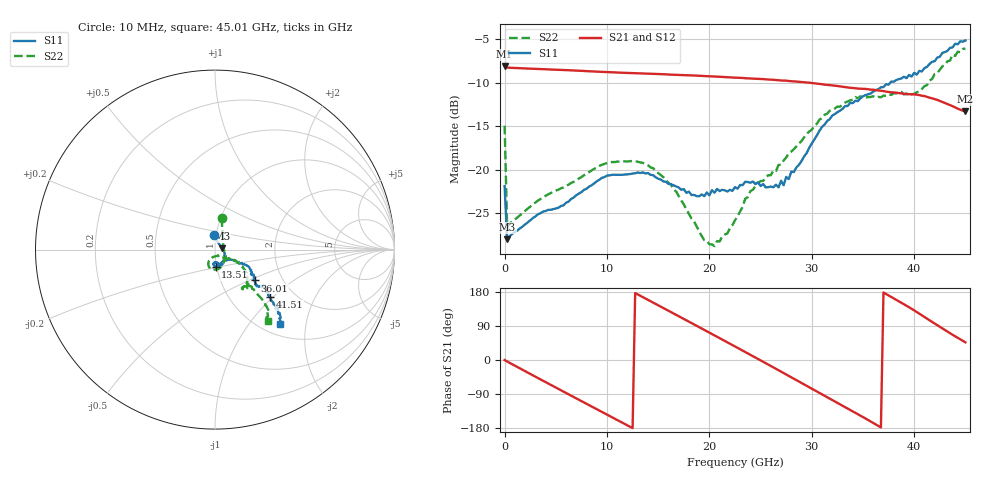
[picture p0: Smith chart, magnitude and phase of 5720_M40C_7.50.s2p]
! Device:  ADRF5720
! Description: 0.5dB LSB GaAs MMIC 6-bit Digital Attenuator
! Frequency:  0.000009 -  40 GHz
! Ports:
!	RF1	= Port 1
!	RF2	= Port 2
! Vdd:  3.3 Volt
! Vss:  -3.3 Volt
! Control:  0/3.3 Volt
! State:  7.50 dB attenuation
! Data:  The device was measured using G-S-G Probes on a matrix board.
!  Data was collected using an calibrated 4 port network analyzer.
!  The reference plane for this measurement is at the launchers.
! Note:  Analog Devices supplies this data as a sample of measured data
!  for this product.  Your particular data for this product may vary.
!  Data was taken at -40 degrees C.
!  Analog Devices reserves the right to change this data at anytime.
# GHZ S DB R 45.0
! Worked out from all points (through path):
!   181 points, 10 MHz to 45.01 GHz, reference 45 ohm
!   highest |S21| = -8.11 dB at 10 MHz (marker M1); lowest = -13.3 dB at 45.01 GHz (marker M2)
!   group delay of S21, straight-line fit = 41.1 ps
!   lowest |S11| = -28.0 dB at 260 MHz (marker M3), VSWR 1.08, Z = 48.7 + j0.651 ohm
!   |S11| at or under -10 dB: start of sweep to 37.68 GHz
!   |S22| runs from -28.8 to -6.1 dB; largest |S21 - S12| = 0.0015
!   S11 on the Smith chart (normalised r, x): 10 MHz: 0.97, +0.16; 13.51 GHz: 0.99, -0.19; 36.01 GHz: 1.45, -0.54; 41.51 GHz: 1.52, -0.96; 45.01 GHz: 1.20, -1.44
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0.01  -21.90 95.5  -8.11 -0.1  -8.13 -0.1  -14.95 78.0
0.26  -28.03 9.7  -8.28 -4.0  -8.30 -4.0  -26.61 7.0
2.26  -26.08 -11.6  -8.39 -33.1  -8.41 -33.2  -24.49 -17.9
4.26  -24.63 -22.1  -8.49 -61.9  -8.51 -61.9  -22.84 -33.1
6.01  -23.81 -36.9  -8.57 -87.0  -8.59 -87.0  -21.84 -47.7
7.76  -22.33 -49.6  -8.67 -112.0  -8.68 -112.1  -20.65 -62.5
10.76  -20.60 -68.7  -8.83 -154.8  -8.85 -154.9  -19.14 -84.5
13.51  -20.32 -88.3  -8.96 166.0  -8.98 165.9  -19.23 -104.2
15.26  -21.14 -94.3  -9.03 140.8  -9.05 140.7  -20.62 -113.5
17.76  -22.67 -93.4  -9.16 104.8  -9.18 104.7  -24.59 -115.8
20.01  -22.96 -86.4  -9.28 72.2  -9.30 72.0  -28.58 -83.9
21.01  -22.47 -82.1  -9.33 57.6  -9.36 57.5  -28.26 -60.5
22.76  -22.19 -78.7  -9.44 32.1  -9.47 32.0  -25.35 -47.2
25.01  -21.89 -62.7  -9.58 -0.9  -9.61 -1.0  -21.31 -35.8
27.26  -21.80 -44.0  -9.77 -34.2  -9.79 -34.4  -18.96 -28.1
30.26  -16.54 -27.6  -10.08 -79.3  -10.11 -79.5  -14.92 -32.6
32.76  -13.23 -28.0  -10.44 -116.9  -10.46 -117.1  -12.78 -40.2
36.01  -11.03 -37.7  -10.82 -166.1  -10.85 -166.3  -11.57 -52.3
37.76  -9.89 -40.4  -11.12 166.5  -11.14 166.3  -11.42 -54.7
39.51  -9.12 -37.1  -11.33 139.2  -11.35 139.0  -11.56 -47.2
41.51  -7.86 -40.7  -11.74 104.8  -11.76 104.5  -9.78 -46.4
45.01  -5.16 -48.8  -13.31 46.6  -13.34 46.5  -6.09 -53.4
